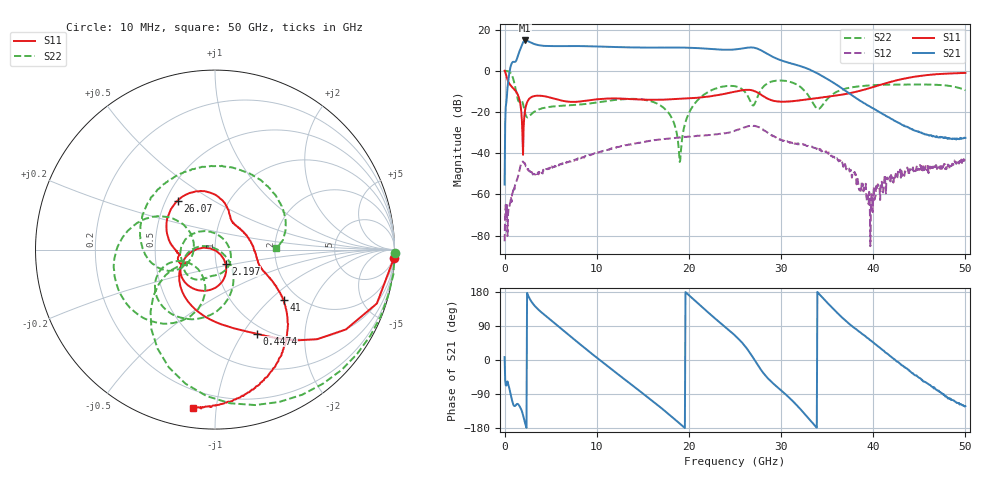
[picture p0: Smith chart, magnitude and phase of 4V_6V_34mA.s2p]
! MARKI MICROWAVE INC.
! Date:  1/07/2020
! Model Number:  APM-6849CH
! Description:  2-port Small Signal S-parameter data for APM-6849CH
! Frequency Range:  10 MHz to 50 GHz
! Port Configuration:  PORT 1: Input
!  PORT 2: Output
! Bias Condition: Vc = +4V, Vb = +6V
! APM-6849CH s2p files are only valid for small signal conditions (below -5 dBm input power)
!S2P File: Measurements: Mag<S11> Ang<S11>, Mag<S21> Ang<S21>, Mag<S12> Ang<S12>, Mag<S22> Ang<S22>!row 1
# Hz S  dB  R 50
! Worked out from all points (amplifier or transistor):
!   801 points, 10 MHz to 50 GHz, reference 50 ohm
!   highest |S21| = 14.8 dB at 2.26 GHz (marker M1)
!   |S21| within 3 dB of that: 1.821 GHz to 10.58 GHz (8.757 GHz wide, 141 % of centre)
!   unconditionally stable (mu >= 1): 116.4 MHz to end of sweep
!   at 8.321 GHz: K = 15.32, MAG = 12.3 dB, |S12| = -42.2 dB
!   at 25 GHz: K = 3.29, MAG = 11.7 dB, |S12| = -29.1 dB
!   at 50 GHz: K = 507.86, MAG = -25.1 dB, |S12| = -42.5 dB
!   S11 on the Smith chart (normalised r, x): 10 MHz: 2, -42; 447.4 MHz: 0.90, -1.16; 2.197 GHz: 1.11, -0.18; 26.07 GHz: 0.57, +0.36; 41 GHz: 1.68, -1.22; 50 GHz: 0.10, -0.87
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1e7  -0.02 -2.7  -55.21 7.7  -82.80 122.4  0.02 -1.0
4.474125e8  -5.64 -63.7  -3.29 -68.2  -66.50 -65.3  -0.36 -51.2
1.5097e9  -12.32 -145.5  8.06 -117.3  -50.40 -73.8  -14.74 -152.0
2.197062e9  -20.17 -53.2  14.69 -163.5  -44.78 -157.1  -19.79 104.3
2.25955e9  -18.36 -58.8  14.76 -169.0  -45.66 -159.5  -20.85 89.6
2.946912e9  -12.68 -100.9  13.52 153.1  -49.13 -176.1  -20.90 -14.2
4.321638e9  -12.34 -139.2  12.11 119.2  -48.09 175.2  -17.98 -61.1
8.383325e9  -14.77 -153.2  12.01 37.9  -42.06 127.0  -16.27 -101.7
1.169516e10  -13.41 -163.2  11.60 -26.0  -37.55 82.5  -14.29 -119.4
1.425715e10  -13.84 -170.8  11.35 -74.1  -35.24 43.7  -13.63 -142.3
1.669416e10  -14.07 -172.3  11.29 -120.6  -33.39 4.6  -16.22 -172.6
1.90062e10  -13.58 -175.5  11.30 -167.6  -32.29 -35.7  -44.27 83.0
2.025595e10  -13.31 -178.3  11.19 165.5  -31.86 -59.0  -18.37 -43.6
2.256799e10  -12.20 173.3  10.54 115.5  -31.03 -105.6  -9.18 -89.3
2.5005e10  -10.09 149.0  10.38 64.5  -29.11 -159.9  -7.47 -138.3
2.606729e10  -9.29 127.4  11.05 37.5  -27.44 166.5  -10.13 -160.7
2.712958e10  -9.86 96.6  11.16 -0.4  -26.69 120.7  -16.06 -118.0
2.844181e10  -13.29 68.7  8.44 -44.8  -29.69 66.9  -6.35 -121.6
3.337832e10  -13.55 6.7  0.05 -164.8  -36.87 -32.2  -14.95 144.3
4.10018e10  -6.48 -36.3  -20.92 26.7  -58.49 47.2  -6.77 139.6
4.168916e10  -5.63 -40.6  -22.62 13.6  -52.72 28.8  -6.71 130.2
5e10  -0.99 -97.8  -32.55 -121.9  -42.49 -84.2  -9.42 1.5
